//Achtung: Parameter BHGIn und BHGOut im FB 1 beachten
//Please note FB 1-parmeter BHGIn, BHGOut

DATA_BLOCK "strdat"		//strdat - ist Anwender DB, is User DB
VERSION : 0.0


  STRUCT
    disp : STRING  [32 ] := '                                ';
		//disp ist Datum fuer Bedienhandgeraet
		//disp is data for the handheld unit
  END_STRUCT ;
BEGIN
END_DATA_BLOCK

